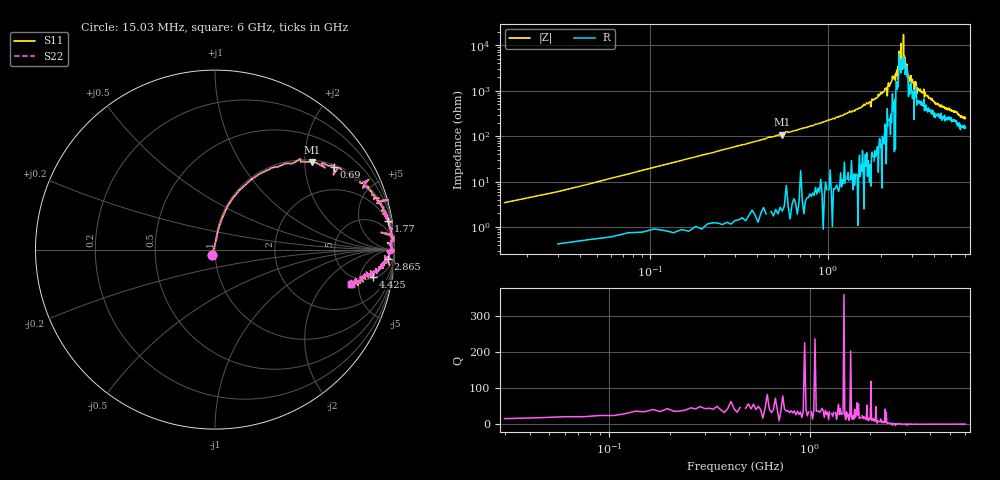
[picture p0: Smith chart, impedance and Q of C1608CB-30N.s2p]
!	Network	Analyzer	HP8753E.07.74:	Oct	30	2002	Serial	No.	JP38451487
!	Hewlett-Packard
!	28	Aug	2009	8:02:50
!	Frequency	S11	S21	S12	S22
#	HZ	S	RI	R	50
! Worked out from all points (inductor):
!   400 points, 15.03 MHz to 6 GHz, reference 50 ohm
!   read as one part in series: L = 31.3 nH near 45.03 MHz
!   highest Q = 43.8 at 555 MHz (marker M1), where L = 31.2 nH
!   self-resonance near 2.55 GHz
!   S11 on the Smith chart (normalised r, x): 15.03 MHz: 0.97, -0.06; 690 MHz: 1.07, +2.84; 1.77 GHz: 2, +12; 2.865 GHz: 16, -26; 4.425 GHz: 5.49, -8.18; 6 GHz: 4.08, -3.96
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1.502992e7  -0.0159 -0.0303  1.02 0.0303  1.02 0.0303  -0.0159 -0.0303
6.00297e7  0.0196 0.116  0.98 -0.116  0.98 -0.116  0.0196 0.116
1.650292e8  0.101 0.289  0.899 -0.289  0.899 -0.289  0.101 0.289
5.550272e8  0.542 0.488  0.458 -0.488  0.458 -0.488  0.542 0.488
6.900266e8  0.664 0.46  0.336 -0.46  0.336 -0.46  0.664 0.46
1.020025e9  0.83 0.361  0.17 -0.361  0.17 -0.361  0.83 0.361
1.770021e9  0.963 0.16  0.0372 -0.16  0.0372 -0.16  0.963 0.16
2.01002e9  0.978 0.112  0.0216 -0.112  0.0216 -0.112  0.978 0.112
2.490018e9  0.986 0.0257  0.0143 -0.0257  0.0143 -0.0257  0.986 0.0257
2.505017e9  0.961 0.0378  0.0387 -0.0378  0.0387 -0.0378  0.961 0.0378
2.535017e9  0.989 0.00684  0.0114 -0.00684  0.0114 -0.00684  0.989 0.00684
2.580017e9  0.981 0.0135  0.0193 -0.0135  0.0193 -0.0135  0.981 0.0135
2.595017e9  0.998 -0.00876  0.00208 0.00876  0.00208 0.00876  0.998 -0.00876
2.655017e9  0.971 -0.01  0.0292 0.01  0.0292 0.01  0.971 -0.01
2.685017e9  0.999 -0.00565  0.00113 0.00565  0.00113 0.00565  0.999 -0.00565
2.700016e9  0.981 -0.00604  0.0186 0.00604  0.0186 0.00604  0.981 -0.00604
2.865016e9  0.965 -0.0541  0.0353 0.0541  0.0353 0.0541  0.965 -0.0541
3.015015e9  0.977 -0.0495  0.0233 0.0495  0.0233 0.0495  0.977 -0.0495
4.00501e9  0.902 -0.132  0.0981 0.132  0.0981 0.132  0.902 -0.132
4.425008e9  0.881 -0.15  0.119 0.15  0.119 0.15  0.881 -0.15
5.010005e9  0.832 -0.151  0.168 0.151  0.168 0.151  0.832 -0.151
6e9  0.755 -0.191  0.245 0.191  0.245 0.191  0.755 -0.191
